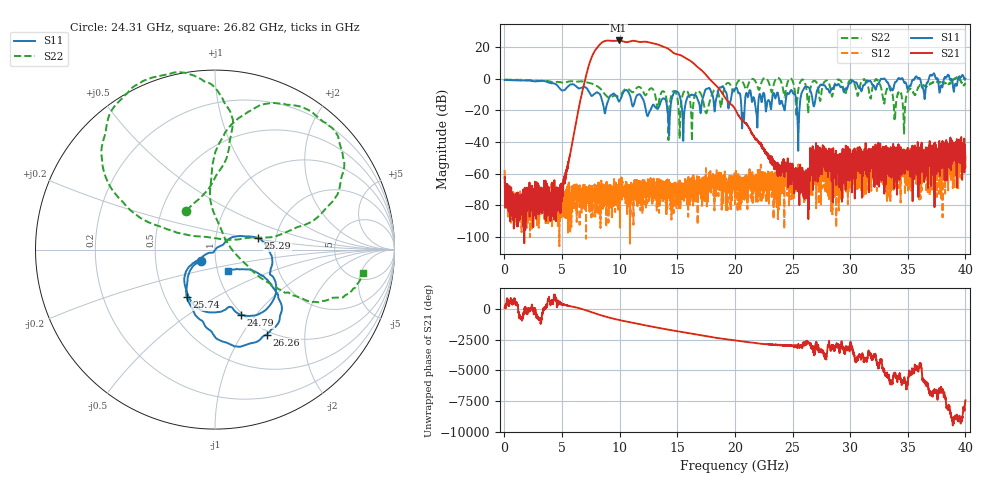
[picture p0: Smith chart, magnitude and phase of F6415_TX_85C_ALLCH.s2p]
!Keysight Technologies,N5245B,MY52451815,A.15.70.20
!Date: Thursday, April 18, 2024 11:15:09
!Correction: S33(C  2-Port  )
!S43(C  2-Port  )
!S34(C  2-Port  )
!S44(C  2-Port  )
!S2P File: Measurements: S33, S43, S34, S44:
# Hz S  RI  R 50
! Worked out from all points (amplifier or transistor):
!   4000 points, 10 MHz to 40 GHz, reference 50 ohm
!   highest |S21| = 24.1 dB at 9.9 GHz (marker M1)
!   |S21| within 3 dB of that: 8.21 GHz to 13.45 GHz (5.243 GHz wide, 48.4 % of centre)
!   unconditionally stable (mu >= 1): start of sweep to 22.47 GHz; 24.86 GHz to 32.68 GHz; 32.98 GHz to 34.13 GHz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
!   at 6.67 GHz: K = 1940.60, MAG = -4.6 dB, |S12| = -73.4 dB
!   at 20.01 GHz: K = 24909.33, MAG = -17.0 dB, |S12| = -79.2 dB
!   at 40 GHz: K = 895.56, MAG = -35.6 dB, |S12| = -49.5 dB
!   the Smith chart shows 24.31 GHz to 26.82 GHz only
!   S11 on the Smith chart (normalised r, x): 24.31 GHz: 0.85, -0.11; 24.79 GHz: 0.98, -0.84; 25.29 GHz: 1.61, +0.22; 25.74 GHz: 0.64, -0.38; 26.26 GHz: 0.95, -1.29; 26.82 GHz: 1.12, -0.27
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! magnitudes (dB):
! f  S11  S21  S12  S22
! 10 MHz  -0.8  -62.8  -57.5  -0.6
! 720 MHz  -1.0  -75.0  -74.2  -0.8
! 4.87 GHz  -6.8  -73.3  -71.6  -2.2
! 6.68 GHz  -5.9  -10.5  -71.6  -1.7
! 7.95 GHz  -8.8  18.7  -71.6  -4.4
! 9.9 GHz  -14.2  24.1  -67.0  -11.1
! 13.34 GHz  -18.5  21.4  -80.1  -17.4
! 16.82 GHz  -14.1  6.9  -68.8  -7.8
! 17.53 GHz  -6.4  2.0  -63.2  -21.6
! 20.01 GHz  -6.6  -19.2  -79.2  -6.3
! 20.69 GHz  -21.6  -26.5  -77.0  -2.4
! 21.17 GHz  -10.5  -30.6  -70.3  -3.4
! 24.31 GHz  -20.0  -59.0  -69.0  -11.4
! 24.79 GHz  -8.1  -53.3  -58.8  0.1
! 25.29 GHz  -12.1  -69.7  -63.6  -16.6
! 25.74 GHz  -10.2  -58.6  -62.5  -1.2
! 26.26 GHz  -5.1  -64.7  -63.6  -10.2
! 26.67 GHz  -10.5  -52.7  -62.1  -3.1
! 26.82 GHz  -17.3  -48.9  -60.2  -1.5
! 33.34 GHz  -3.6  -59.6  -52.3  -4.9
! 34.67 GHz  -2.1  -47.5  -57.1  -33.9
! 40 GHz  -0.1  -55.6  -49.5  -2.9
